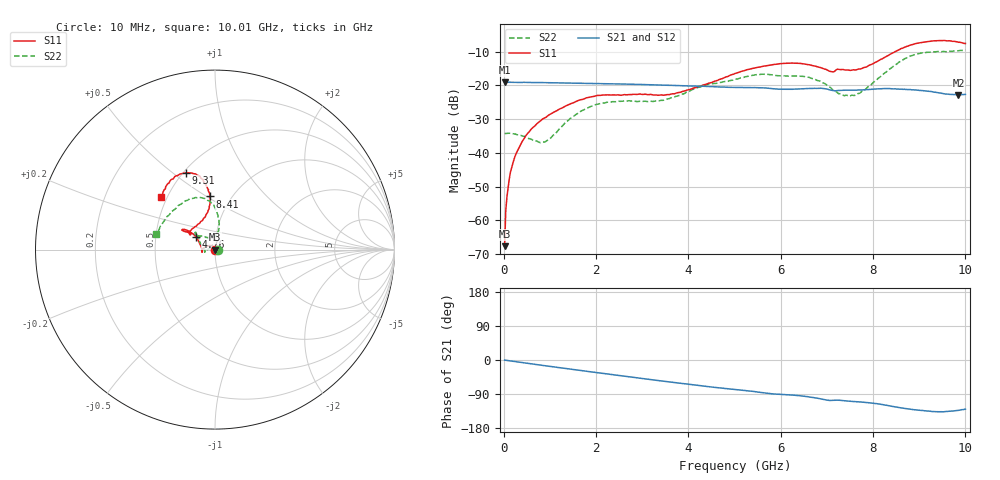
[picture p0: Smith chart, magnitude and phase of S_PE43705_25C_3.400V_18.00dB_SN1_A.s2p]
! Device ID: PE43705
! Serial: 1
! Insertion: A
! Impedance: 50 ohm
! Temp: 25C
! VDD: 3.400V
! Attenuation Step: 18.00dB
#  Hz  S  RI  R  50
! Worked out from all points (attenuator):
!   401 points, 10 MHz to 10.01 GHz, reference 50 ohm
!   highest |S21| = -19.03 dB at 10 MHz (marker M1); lowest = -22.8 dB at 9.86 GHz (marker M2)
!   lowest |S11| = -67.6 dB at 10 MHz (marker M3), VSWR 1.00, Z = 50 + j0.0407 ohm
!   |S11| at or under -10 dB: start of sweep to 8.48 GHz
!   |S22| runs from -36.9 to -9.5 dB; largest |S21 - S12| = 0.0012
!   S11 on the Smith chart (normalised r, x): 10 MHz: 1.00, +0.00; 4.76 GHz: 0.80, +0.12; 8.41 GHz: 0.79, +0.52; 9.31 GHz: 0.51, +0.56; 10.01 GHz: 0.46, +0.33
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1e7  -8.41e-05 0.000407  0.1119 -0.000473  0.1119 -0.000452  0.0193 0.000282
8.5e7  0.000112 0.00299  0.1115 -0.00304  0.1115 -0.003  0.0195 0.00196
1.6e8  -0.000381 0.00597  0.1114 -0.00557  0.1113 -0.00547  0.0189 0.00415
2.6e8  -0.00165 0.00968  0.1108 -0.0089  0.1107 -0.0088  0.0175 0.00694
4.1e8  -0.00476 0.0147  0.1107 -0.0132  0.1103 -0.0138  0.0145 0.0104
8.85e8  -0.0246 0.0223  0.1064 -0.0286  0.1063 -0.0285  -0.00454 0.0138
1.685e9  -0.0612 0.00921  0.0953 -0.0507  0.0952 -0.0508  -0.0423 6.77e-05
2.26e9  -0.0719 -0.0086  0.0843 -0.0644  0.0844 -0.0642  -0.0552 -0.0122
3.36e9  -0.0716 -0.00485  0.0591 -0.0828  0.059 -0.0826  -0.0589 0.00211
4.76e9  -0.1064 0.0727  0.0252 -0.0913  0.0253 -0.0911  -0.0927 0.0655
5.01e9  -0.1222 0.0879  0.0198 -0.0916  0.0199 -0.0916  -0.0989 0.0741
5.985e9  -0.1776 0.1127  -0.000911 -0.088  -0.000339 -0.0879  -0.1056 0.0906
6.685e9  -0.1698 0.1007  -0.0138 -0.0893  -0.0135 -0.0893  -0.0984 0.0796
7.11e9  -0.1345 0.0865  -0.0245 -0.0812  -0.0244 -0.0814  -0.0546 0.0702
7.535e9  -0.0993 0.136  -0.0279 -0.0803  -0.0276 -0.0804  -0.00959 0.0709
7.785e9  -0.0659 0.1695  -0.0311 -0.08  -0.0309 -0.0805  0.00782 0.0838
8.36e9  -0.0266 0.2846  -0.046 -0.0774  -0.0458 -0.0771  0.0198 0.1731
8.41e9  -0.0297 0.2963  -0.0474 -0.0757  -0.0475 -0.0761  0.0168 0.1828
8.835e9  -0.0719 0.3925  -0.0559 -0.0659  -0.0551 -0.0663  -0.0365 0.2725
9.31e9  -0.1633 0.4279  -0.0577 -0.0558  -0.0577 -0.0562  -0.1442 0.2806
9.86e9  -0.2761 0.3384  -0.0493 -0.0531  -0.0496 -0.053  -0.2907 0.1491
1.001e10  -0.2989 0.2938  -0.0473 -0.0567  -0.0484 -0.0567  -0.3261 0.0845
